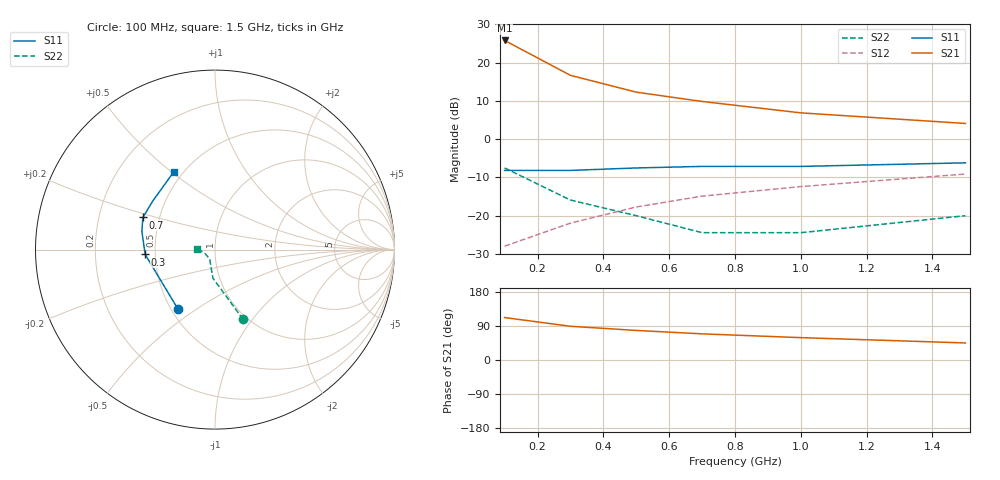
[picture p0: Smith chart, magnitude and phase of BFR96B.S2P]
! SCCS file tdata/motorola: @(#)get -r1.1 /eesof/src/tdata/motorola/s.bfr96b.s2p # Version date: 10/22/90
!  BFR96B.S2P
!  BFR96
!  VCE=5V; IC=25mA
#  GHZ S MA R 50
!  S-PARAMETER DATA
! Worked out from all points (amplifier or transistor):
!   6 points, 100 MHz to 1.5 GHz, reference 50 ohm
!   highest |S21| = 25.8 dB at 100 MHz (marker M1)
!   |S21| within 3 dB of that: start of sweep to 165.9 MHz
!   unconditionally stable (mu >= 1): 293.9 MHz to 1.493 GHz
!   at 300 MHz: K = 1.01, MAG = 18.8 dB, |S12| = -21.9 dB
!   at 700 MHz: K = 1.00, MAG = 12.0 dB, |S12| = -14.9 dB
!   at 1.5 GHz: K = 1.00, MSG = 6.6 dB, |S12| = -9.1 dB
!   S11 on the Smith chart (normalised r, x): 100 MHz: 0.54, -0.42; 300 MHz: 0.44, -0.03; 700 MHz: 0.40, +0.18; 1.5 GHz: 0.45, +0.51
0.1  0.39 -122.0  19.4 112.0  0.04 60.0  0.42 -68.0
0.3  0.39 -176.0  6.8 89.0  0.08 68.0  0.16 -94.0
0.5  0.42 166.0  4.1 78.0  0.13 70.0  0.1 -103.0
0.7  0.44 156.0  3.1 69.0  0.18 68.0  0.06 -119.0
1  0.44 142.0  2.2 59.0  0.24 64.0  0.06 -159.0
1.5  0.49 118.0  1.6 45.0  0.35 57.0  0.1 177.0
